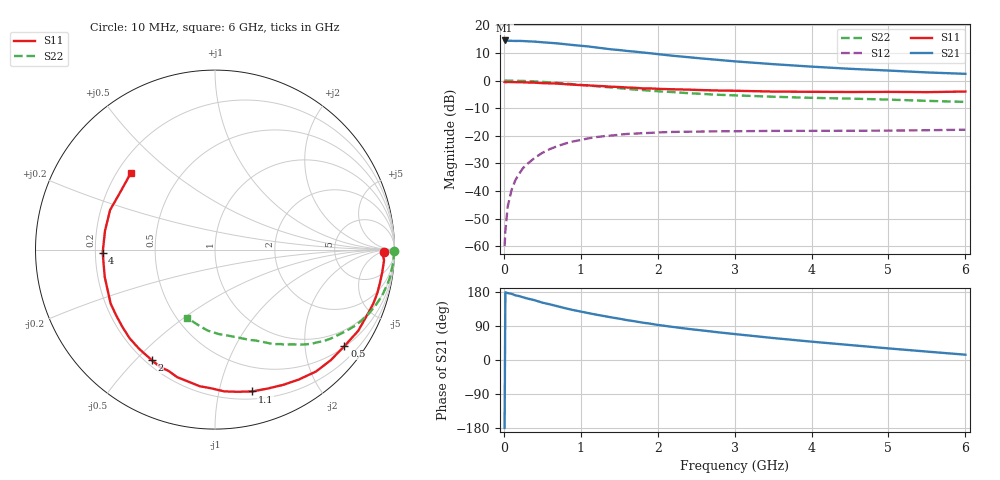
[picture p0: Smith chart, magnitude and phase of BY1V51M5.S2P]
! SIEMENS Small Signal Semiconductors
! BFY420
! Si NPN RF SIEGET Grounded Emitter Transistor in MICRO-X
! VCE = 1.5 V  IC = 1.5 mA
! Common Emitter S-Parameters:  October  1996
# GHz  S  MA  R  50
!  f  S11  S21  S12  S22
! GHz  MAG  ANG  MAG  ANG  MAG  ANG  MAG  ANG
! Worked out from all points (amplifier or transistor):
!   36 points, 10 MHz to 6 GHz, reference 50 ohm
!   highest |S21| = 14.5 dB at 10 MHz (marker M1)
!   |S21| within 3 dB of that: start of sweep to 1.334 GHz
!   unconditionally stable (mu >= 1): 4.245 GHz to end of sweep
!   at 250 MHz: K = 0.05, MSG = 23.0 dB, |S12| = -31.7 dB
!   at 1.4 GHz: K = 0.26, MSG = 15.6 dB, |S12| = -19.9 dB
!   at 6 GHz: K = 1.28, MAG = 6.9 dB, |S12| = -17.8 dB
!   S11 on the Smith chart (normalised r, x): 10 MHz: 32, -7; 500 MHz: 0.52, -2.93; 1.1 GHz: 0.27, -1.26; 2 GHz: 0.23, -0.56; 4 GHz: 0.23, -0.01; 6 GHz: 0.26, +0.36
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0.01  0.9418 -0.7  5.337 -179.3  0.001 98.8  0.9986 -0.4
0.02  0.9335 -1.4  5.31 178.6  0.0019 89.4  0.9993 -0.8
0.05  0.9438 -3.6  5.253 176.6  0.0052 93.7  0.9965 -1.9
0.1  0.9403 -7.6  5.256 174.6  0.0104 86.7  0.996 -4.0
0.15  0.9376 -11.1  5.226 170.7  0.0157 83.1  0.9916 -5.8
0.25  0.9321 -18.7  5.21 165.5  0.026 78.1  0.9853 -9.7
0.4  0.9172 -29.6  5.086 157.8  0.0398 72.4  0.9656 -15.4
0.5  0.8995 -36.7  4.947 151.4  0.049 68.5  0.9479 -19.0
0.6  0.892 -43.7  4.839 146.8  0.0576 64.1  0.9287 -22.5
0.8  0.8616 -57.1  4.559 136.6  0.0725 56.0  0.8841 -29.0
1.1  0.8171 -75.3  4.155 123.7  0.0899 46.4  0.8142 -37.4
1.4  0.7736 -91.4  3.676 112.4  0.1011 38.0  0.7507 -44.4
1.6  0.7494 -101.9  3.446 105.2  0.1079 33.4  0.7084 -48.4
2  0.7095 -119.7  3.02 92.6  0.1149 25.7  0.6416 -55.1
2.2  0.6962 -127.3  2.816 87.2  0.1176 22.2  0.6192 -58.3
2.4  0.6857 -134.0  2.653 82.0  0.1186 19.7  0.5913 -61.2
2.8  0.6609 -146.7  2.364 72.8  0.1207 15.2  0.5522 -66.3
3.5  0.633 -166.1  1.986 58.0  0.1227 9.7  0.5101 -74.5
4  0.6261 -178.5  1.791 48.4  0.1229 6.9  0.4872 -80.6
4.5  0.6218 170.2  1.635 39.5  0.1233 4.8  0.4717 -87.2
5.5  0.6176 147.8  1.406 22.2  0.1261 2.7  0.4295 -103.0
6  0.6338 137.9  1.326 14.0  0.1289 2.5  0.411 -112.2
